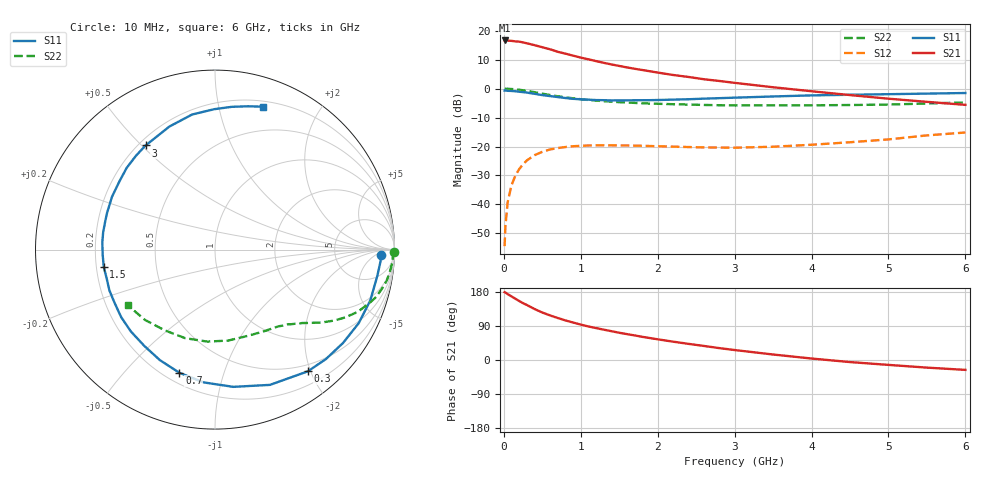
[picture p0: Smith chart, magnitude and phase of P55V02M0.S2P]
! SIEMENS Small Signal Semiconductors
! BFP183
! Si NPN RF Bipolar Junction Transistor in SOT143
! VCE = 5 V  IC = 2 mA
! Common Emitter S-Parameters:  March  1996
# GHz  S  MA  R  50
!  f  S11  S21  S12  S22
! GHz  MAG  ANG  MAG  ANG  MAG  ANG  MAG  ANG
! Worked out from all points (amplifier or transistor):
!   36 points, 10 MHz to 6 GHz, reference 50 ohm
!   highest |S21| = 16.6 dB at 10 MHz (marker M1)
!   |S21| within 3 dB of that: start of sweep to 594.5 MHz
!   unconditionally stable (mu >= 1): 2.142 GHz to 5.846 GHz
!   at 250 MHz: K = 0.12, MSG = 21.0 dB, |S12| = -26.1 dB
!   at 1.4 GHz: K = 0.67, MSG = 14.0 dB, |S12| = -19.6 dB
!   at 6 GHz: K = 0.97, MSG = 4.8 dB, |S12| = -15.2 dB
!   S11 on the Smith chart (normalised r, x): 10 MHz: 23, -9; 300 MHz: 0.39, -1.96; 700 MHz: 0.26, -0.72; 1.5 GHz: 0.23, -0.07; 3 GHz: 0.23, +0.51; 6 GHz: 0.25, +1.36
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0.01  0.9255 -1.7  6.783 179.0  0.0019 87.8  0.9997 -0.7
0.02  0.9247 -4.0  6.771 178.0  0.0042 86.5  0.99 -1.3
0.05  0.9161 -9.3  6.746 173.8  0.011 86.4  0.9926 -3.4
0.1  0.9103 -18.1  6.671 167.7  0.0215 78.2  0.9835 -6.8
0.2  0.8828 -36.1  6.465 155.6  0.0408 69.5  0.9554 -13.2
0.25  0.8683 -44.6  6.269 149.9  0.0493 64.9  0.9354 -16.4
0.3  0.8529 -52.7  6.055 145.1  0.0577 60.5  0.9116 -19.0
0.4  0.8135 -67.9  5.625 134.4  0.0709 52.5  0.8672 -23.6
0.5  0.7715 -82.4  5.175 125.3  0.0809 45.9  0.8179 -27.5
0.6  0.7425 -95.0  4.781 117.7  0.0889 40.0  0.7754 -30.6
0.7  0.7144 -106.1  4.323 110.9  0.0939 35.2  0.7373 -33.1
0.9  0.6658 -126.2  3.709 98.9  0.1011 27.5  0.6795 -36.9
1.1  0.6442 -144.2  3.205 88.4  0.1042 21.7  0.6352 -40.1
1.3  0.6309 -158.8  2.784 80.0  0.105 17.4  0.6061 -43.0
1.5  0.6275 -171.2  2.462 71.9  0.1044 14.5  0.5827 -45.5
1.8  0.6305 171.2  2.095 61.1  0.1029 11.9  0.558 -49.8
2.2  0.645 152.8  1.719 48.4  0.0995 10.2  0.5375 -56.0
3  0.6973 123.7  1.257 26.3  0.0954 13.6  0.5124 -71.1
3.5  0.7313 110.3  1.055 14.5  0.0991 17.9  0.5121 -81.8
4.5  0.7824 90.3  0.773 -5.5  0.1185 24.1  0.5206 -108.6
5.5  0.8196 77.0  0.591 -20.1  0.1556 24.7  0.553 -134.9
6  0.8391 71.6  0.524 -26.1  0.1746 21.3  0.5767 -147.5
